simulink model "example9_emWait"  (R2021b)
settings: Solver=FixedStepAuto  StartTime=0  StopTime=inf  FixedStep=0.5  RelTol=1e-3  EnableMultiTasking=on
undefined symbols (not defined in the file or in its folder): based, classic, dsPic33, MCC, Microchip, PIC24
libraries: embeddedCreatorLib x2, emMBSlaveLib x1

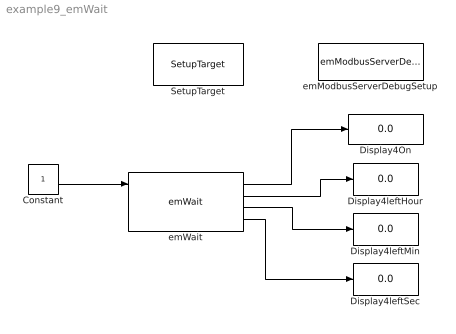
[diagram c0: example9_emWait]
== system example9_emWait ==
  Constant : Constant  OutDataTypeStr=boolean
  Display4On : Display
  Display4leftHour : Display
  Display4leftMin : Display
  Display4leftSec : Display
  SetupTarget : embeddedCreatorLib/SetupTarget  Tag=SetupTarget  Priority=0  c_platform=Microchip PIC24/dsPic33 based on MCC classic  c_debug=on
  emModbusServerDebugSetup : emMBSlaveLib/emModbusServerDebugSetup  Tag=emModbusSlaveSetup  c_objID=0  c_uartNo=2  c_baudrate=19200  c_serverID=1  c_baudrate4PC=19200  c_forceLongerSpace=on  c_holdingRegsQTY=1000  c_minHoldingAddr=789  c_inputRegsQTY=200  c_minInputRegAddr=20  c_coilRegsQTY=300  c_minCoilAddr=30  c_discreteRegsQTY=400  c_minDiscreteAddr=40  c_enableDebug=on  c_breakpointMaxQTY=100  c_probeMaxWordQTY=200  c_emWaitQTY=1  g_COMPortNo=COM5  c_Name_method=By physical port name and bit number  c_PortName=B  c_BitNo=11  c_TxEnable485="\"LATBbits.LATB11\""  c_TxEnable485Polarity=on
  emWait : embeddedCreatorLib/emWait  Tag=emWait  c_hours=0  c_minutes=1  c_seconds=12  c_ms=2  c_ObjID=0  c_serverID=1  c_UartNo=2  c_sampleTime=-1
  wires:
  emWait/1 -> Display4On/1
  emWait/2 -> Display4leftHour/1
  emWait/3 -> Display4leftMin/1
  emWait/4 -> Display4leftSec/1
  Constant/1 -> emWait/1
